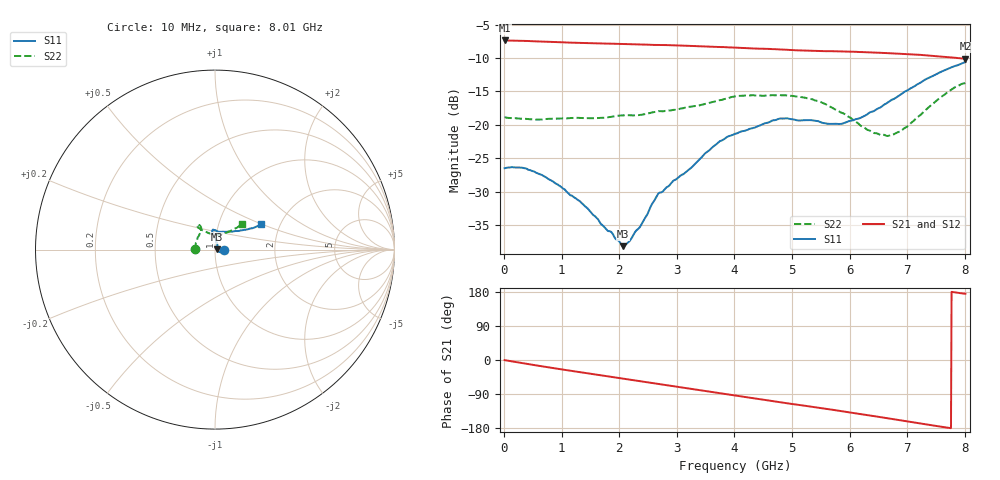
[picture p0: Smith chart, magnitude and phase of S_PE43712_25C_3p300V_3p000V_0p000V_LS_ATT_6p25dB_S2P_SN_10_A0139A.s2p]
! DEVICE ID: PE43712
! File Path: z:\PE43713\PE43713_CHAR_NOM_04292014\AMB\3p300\LS_ATT_6p25dB\PE43713_AMB_3p300V_3p000V_0p000V_LS_ATT_6p25dB_S2P_SN_10_A0139A.s2p
! Serial: 10
! Lot: A0139A
! Temp: 25C
! VDD: 3.300
! VSS: 0.000
! Control_Hi: 3.000
! Control_Lo: 0.000
! Attenuation Step: 6.25dB
! Port 1: RF1
! Port 2: RF2
! ThroughPath:1-2
! IDD: 0.0001470468
! ISS: -9.47e-008
#  Hz  S  RI  R  50
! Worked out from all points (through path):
!   801 points, 10 MHz to 8.01 GHz, reference 50 ohm
!   highest |S21| = -7.38 dB at 10 MHz (marker M1); lowest = -10.1 dB at 8.01 GHz (marker M2)
!   group delay of S21, straight-line fit = 63.6 ps
!   lowest |S11| = -38.1 dB at 2.07 GHz (marker M3), VSWR 1.03, Z = 51.2 + j0.276 ohm
!   |S11| at or under -10 dB: start of sweep to end of sweep
!   |S22| runs from -21.7 to -13.7 dB; largest |S21 - S12| = 0.0014
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1e7  0.0474 -9.14e-05  0.4277 -0.00248  0.4275 -0.00232  -0.114 0.000662
3.3e8  0.0469 -0.00896  0.4193 -0.0634  0.4189 -0.0629  -0.1107 0.00977
6.3e8  0.0403 -0.0137  0.4038 -0.1155  0.4038 -0.1155  -0.1082 0.0181
9.6e8  0.0318 -0.0149  0.3796 -0.1678  0.3798 -0.1678  -0.108 0.0277
1.35e9  0.0227 -0.0125  0.3445 -0.222  0.3445 -0.2221  -0.1056 0.0392
2.07e9  0.0121 0.00269  0.2626 -0.3051  0.2626 -0.305  -0.0975 0.0663
2.17e9  0.0123 0.00536  0.2496 -0.3146  0.2496 -0.3145  -0.0954 0.0696
2.36e9  0.0117 0.0127  0.2234 -0.3313  0.2234 -0.3312  -0.0893 0.078
2.68e9  0.0137 0.0275  0.1781 -0.353  0.1781 -0.3531  -0.0806 0.0977
3.24e9  0.00546 0.047  0.0927 -0.378  0.0928 -0.3781  -0.0777 0.1124
3.71e9  0.000842 0.0732  0.0204 -0.3817  0.0202 -0.3818  -0.08 0.1286
4.01e9  -0.0053 0.0855  -0.0251 -0.3774  -0.0251 -0.3774  -0.0886 0.1371
4.79e9  -0.0128 0.1109  -0.1332 -0.3413  -0.1332 -0.3416  -0.098 0.1354
5.35e9  -0.000239 0.1081  -0.1981 -0.2982  -0.1981 -0.298  -0.0948 0.1232
5.63e9  0.0128 0.101  -0.2268 -0.2739  -0.2268 -0.2741  -0.0801 0.1133
5.87e9  0.0267 0.0984  -0.252 -0.2497  -0.2515 -0.2497  -0.0634 0.1052
6.18e9  0.0531 0.099  -0.278 -0.2135  -0.2775 -0.2135  -0.0372 0.0922
6.4e9  0.0757 0.1003  -0.2934 -0.1864  -0.2929 -0.1863  -0.0179 0.086
6.68e9  0.1088 0.102  -0.3091 -0.1491  -0.3088 -0.1491  0.0114 0.0822
6.9e9  0.1346 0.1041  -0.3186 -0.119  -0.3183 -0.119  0.0333 0.0843
7.7e9  0.2288 0.1274  -0.321 -0.00788  -0.3207 -0.0082  0.1248 0.1244
8.01e9  0.2589 0.1404  -0.3107 0.0288  -0.3101 0.0282  0.1499 0.1411
